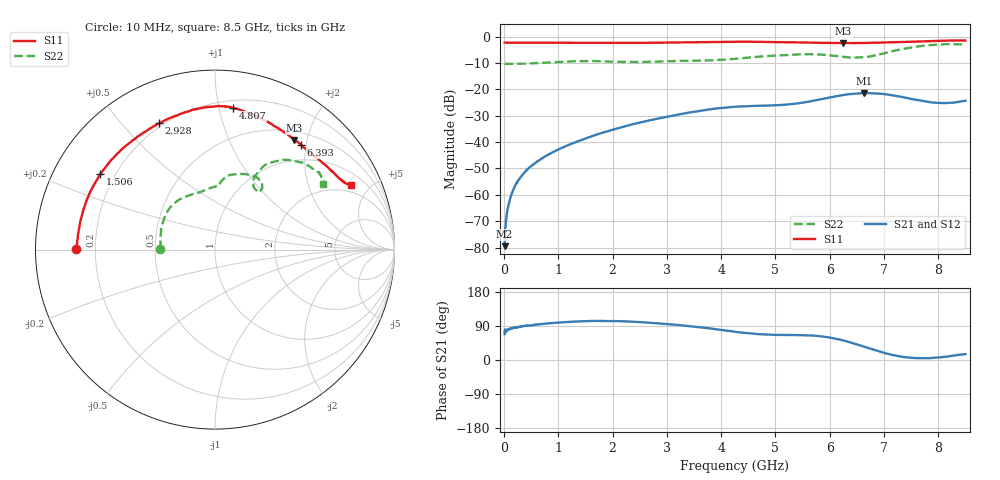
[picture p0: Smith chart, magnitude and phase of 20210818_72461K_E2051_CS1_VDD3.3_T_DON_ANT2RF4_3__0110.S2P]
!Agilent Technologies,E5071C,MY46417908,A.11.23
!Date: Wed Aug 18 14:33:30 2021
!Data & Calibration Information:
!Freq	S11:SOLT2(ON)	S21:SOLT2(ON)	S12:SOLT2(ON)	S22:SOLT2(ON)
!PortZ  Port1:50+j0  Port2:50+j0
!Above PortZ is port z conversion or system Z0 setting when saving the data.
!When reading, reference impedance value at option line is always used.
# Hz S dB R 50
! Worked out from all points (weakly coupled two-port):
!   1601 points, 10 MHz to 8.5 GHz, reference 50 ohm
!   highest |S21| = -21.44 dB at 6.638 GHz (marker M1); lowest = -79.5 dB at 10 MHz (marker M2)
!   lowest |S11| = -2.5 dB at 6.25 GHz (marker M3), VSWR 7.10, Z = 31.7 + j89.3 ohm
!   |S11| at or under -10 dB: nowhere
!   |S22| runs from -10.3 to -2.8 dB; largest |S21 - S12| = 0.0004
!   S11 on the Smith chart (normalised r, x): 10 MHz: 0.13, +0.00; 1.506 GHz: 0.15, +0.29; 2.928 GHz: 0.18, +0.64; 4.807 GHz: 0.26, +1.10; 6.393 GHz: 0.70, +1.91; 8.5 GHz: 1.54, +3.84
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1e7  -2.24 179.7  -79.47 68.0  -77.14 73.3  -10.30 179.6
6.30625e7  -2.27 178.5  -65.90 79.1  -65.85 78.7  -10.32 178.2
1.108188e8  -2.28 177.4  -61.47 82.1  -61.34 81.5  -10.32 176.9
2.01025e8  -2.29 175.3  -56.56 85.9  -56.77 85.1  -10.32 174.5
3.28375e8  -2.30 172.5  -52.64 88.7  -52.69 88.4  -10.25 171.4
4.875625e8  -2.31 168.8  -49.29 91.1  -49.28 91.4  -10.15 167.6
7.422625e8  -2.32 163.1  -45.61 95.5  -45.58 95.8  -9.89 159.8
1.426769e9  -2.34 148.5  -39.17 102.1  -39.18 102.2  -9.29 135.4
1.506362e9  -2.34 146.7  -38.59 102.5  -38.60 102.6  -9.29 132.6
2.196175e9  -2.36 131.3  -34.19 102.1  -34.19 102.1  -9.58 111.0
2.843538e9  -2.29 115.7  -31.02 96.5  -31.02 96.4  -9.45 98.6
2.928438e9  -2.28 113.8  -30.73 95.6  -30.72 95.5  -9.36 97.3
4.255e9  -1.96 89.9  -26.58 74.6  -26.59 74.5  -8.43 85.2
4.80685e9  -1.99 82.7  -26.19 67.2  -26.18 67.3  -7.43 78.2
5.671769e9  -2.27 67.6  -24.43 64.7  -24.44 64.8  -6.68 58.8
6.25015e9  -2.46 54.1  -22.18 51.5  -22.20 51.5  -7.64 52.5
6.393419e9  -2.44 50.6  -21.76 45.8  -21.78 45.7  -7.95 52.9
6.637506e9  -2.39 44.7  -21.44 34.9  -21.47 34.8  -7.78 57.9
7.088538e9  -2.16 35.8  -22.04 15.6  -22.07 15.4  -5.86 60.5
7.60855e9  -1.87 28.5  -24.04 5.0  -24.05 4.9  -3.77 50.3
8.080806e9  -1.56 25.8  -25.19 7.7  -25.17 7.7  -2.92 37.6
8.5e9  -1.49 25.5  -24.33 15.5  -24.35 15.3  -3.04 31.0
